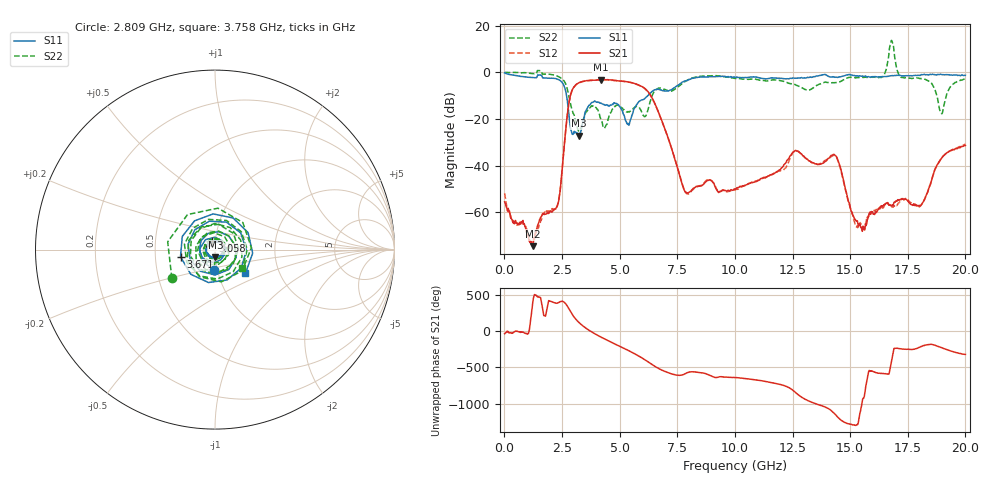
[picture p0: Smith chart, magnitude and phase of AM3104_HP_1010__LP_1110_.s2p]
!Created with skrf (http://scikit-rf.org).
# Hz S RI R 50.0
!freq ReS11 ImS11 ReS21 ImS21 ReS12 ImS12 ReS22 ImS22
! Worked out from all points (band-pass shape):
!   1601 points, 10 MHz to 20 GHz, reference 50 ohm
!   highest |S21| = -3.18 dB at 4.183 GHz (marker M1); lowest = -74.5 dB at 1.234 GHz (marker M2)
!   |S21| within 3 dB of the highest: 3.032 GHz to 5.977 GHz (2.945 GHz wide, 65.4 % of centre)
!   lowest |S11| = -27.2 dB at 3.233 GHz (marker M3), VSWR 1.09, Z = 50 - j4.37 ohm
!   |S11| at or under -10 dB: 2.698 GHz to 6.227 GHz (3.53 GHz wide, 79.1 % of centre)
!   |S22| runs from -25.4 to 13.6 dB; largest |S21 - S12| = 0.077
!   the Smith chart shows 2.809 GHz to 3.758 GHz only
!   S11 on the Smith chart (normalised r, x): 2.809 GHz: 0.96, -0.22; 3.058 GHz: 0.97, +0.09; 3.671 GHz: 0.68, -0.06; 3.758 GHz: 1.35, -0.37
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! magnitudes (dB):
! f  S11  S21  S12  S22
! 10 MHz  -0.3  -55.6  -51.9  -0.1
! 1.234 GHz  -2.3  -74.5  -71.7  -0.5
! 2.309 GHz  -3.0  -56.8  -57.1  -1.7
! 2.809 GHz  -19.0  -12.7  -12.7  -10.8
! 3.058 GHz  -26.0  -5.8  -5.8  -20.0
! 3.233 GHz  -27.2  -4.5  -4.6  -25.4
! 3.346 GHz  -24.4  -4.1  -4.2  -23.4
! 3.671 GHz  -14.1  -3.6  -3.6  -15.2
! 3.758 GHz  -13.4  -3.5  -3.5  -14.8
! 4.183 GHz  -13.3  -3.2  -3.2  -20.1
! 5.37 GHz  -22.1  -4.2  -4.2  -16.8
! 6.682 GHz  -7.3  -17.0  -17.1  -6.8
! 7.894 GHz  -3.7  -51.7  -51.9  -3.7
! 10.01 GHz  -2.2  -50.3  -50.4  -2.7
! 12.6 GHz  -2.6  -33.7  -33.7  -5.2
! 13.34 GHz  -2.2  -38.7  -38.7  -7.1
! 14.37 GHz  -2.1  -35.8  -36.1  -4.4
! 15.54 GHz  -1.6  -67.8  -66.1  -2.2
! 16.68 GHz  -1.6  -56.8  -56.9  7.3
! 18.03 GHz  -1.4  -57.2  -57.5  -2.7
! 18.95 GHz  -0.9  -37.1  -36.9  -17.5
! 20 GHz  -1.3  -31.4  -30.9  -2.9
